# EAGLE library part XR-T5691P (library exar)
T1 receive BUFFER
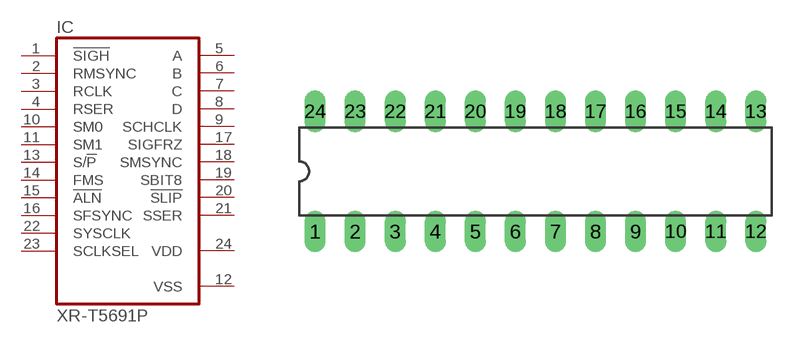
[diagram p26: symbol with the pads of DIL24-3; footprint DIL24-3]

Designator prefix IC

## XR-T5691P (OC_FARNELL: unknown; OC_NEWARK: unknown)  [DIL24-3]
1  !SIGH  in
2  RMSYNC  in
3  RCLK  in
4  RSER  in
5  A  out
6  B  out
7  C  out
8  D  out
9  SCHCLK  out
10  SM0  in
11  SM1  in
12  VSS  pwr
13  S/!P  in
14  FMS  in
15  !ALN  in
16  SFSYNC  in
17  SIGFRZ  out
18  SMSYNC  out
19  SBIT8  out
20  !SLIP  out
21  SSER  out
22  SYSCLK  in
23  SCLKSEL  in
24  VDD  pwr

## Footprint DIL24-3 (pad centres in mm)
Dual In Line Package 0.3 inch
drill 0.813 long: 1 -13.97,-3.81; 2 -11.43,-3.81; 3 -8.89,-3.81; 4 -6.35,-3.81; 5 -3.81,-3.81; 6 -1.27,-3.81; 7 1.27,-3.81; 8 3.81,-3.81; 9 6.35,-3.81; 10 8.89,-3.81; 11 11.43,-3.81; 12 13.97,-3.81; 13 13.97,3.81; 14 11.43,3.81; 15 8.89,3.81; 16 6.35,3.81; 17 3.81,3.81; 18 1.27,3.81; 19 -1.27,3.81; 20 -3.81,3.81; 21 -6.35,3.81; 22 -8.89,3.81; 23 -11.43,3.81; 24 -13.97,3.81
